(* Logix 5000 Rung export; software revision 20.03 *)

TYPE CONTROL_OUT_1 :
STRUCT
   TriggerEnable : BOOL;
   Trigger : BOOL;
   BufferResultsEnable : BOOL;
   InspectionResultsAck : BOOL;
   ExecuteCommand : BOOL;
   Reserved0_5 : BOOL;
   Reserved0_6 : BOOL;
   SetOffline : BOOL;
   Reserved_Byte1 : SINT;
   SetUserData : BOOL;
   Reserved2_1 : BOOL;
   ClearError : BOOL;
   ClearExposureComplete : BOOL;
   Reserved2_4 : BOOL;
   Reserved2_5 : BOOL;
   Reserved2_6 : BOOL;
   Reserved2_7 : BOOL;
   ExternalEvent0 : BOOL;
   ExternalEvent1 : BOOL;
   ExternalEvent2 : BOOL;
   ExternalEvent3 : BOOL;
   ExternalEvent4 : BOOL;
   ExternalEvent5 : BOOL;
   ExternalEvent6 : BOOL;
   ExternalEvent7 : BOOL;
   CommandID : INT;
   Reserved_Bytes6and7 : INT;
END_STRUCT
END_TYPE

TYPE INSIGHT_IN_1 :
STRUCT
   Status : STATUS_IN_1;
   InspectionResults : SINT[484];
END_STRUCT
END_TYPE

TYPE STATUS_IN_1 :
STRUCT
   TriggerReady : BOOL;
   TriggerAck : BOOL;
   Reserved0_2 : BOOL;
   AcqError : BOOL;
   OfflineReason0 : BOOL;
   OfflineReason1 : BOOL;
   OfflineReason2 : BOOL;
   Online : BOOL;
   Reserved1_0 : BOOL;
   InspectionCompleted : BOOL;
   ResultsBufferOverrun : BOOL;
   ResultsValid : BOOL;
   CommandExecuting : BOOL;
   CommandCompleted : BOOL;
   CommandFailed : BOOL;
   Error : BOOL;
   SetUserDataAck : BOOL;
   Reserved2_1 : BOOL;
   Reserved2_2 : BOOL;
   ExposureComplete : BOOL;
   JobPass : BOOL;
   TestRunReady : BOOL;
   Reserved2_6 : BOOL;
   Reserved2_7 : BOOL;
   ExternalEventAck0 : BOOL;
   ExternalEventAck1 : BOOL;
   ExternalEventAck2 : BOOL;
   ExternalEventAck3 : BOOL;
   ExternalEventAck4 : BOOL;
   ExternalEventAck5 : BOOL;
   ExternalEventAck6 : BOOL;
   ExternalEventAck7 : BOOL;
   ErrorID : INT;
   CommandResultCode : INT;
   CurrentJobID : INT;
   AcquisitionID : INT;
   InspectionID : INT;
   InspectionResultCode : INT;
END_STRUCT
END_TYPE

TYPE INSIGHT_OUT_1 :
STRUCT
   Control : CONTROL_OUT_1;
   UserData : SINT[488];
END_STRUCT
END_TYPE

VAR_GLOBAL   (* controller tags *)
   insight1_in : INSIGHT_IN_1;
   insight1_out : INSIGHT_OUT_1;
END_VAR

PROGRAM MainProgram

ROUTINE MainRoutine   (* ladder *)
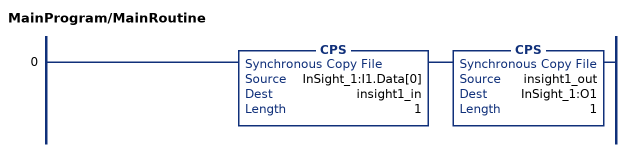
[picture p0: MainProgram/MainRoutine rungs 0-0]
   0: CPS(InSight_1:I1.Data[0],insight1_in,1)CPS(insight1_out,InSight_1:O1,1);
END_ROUTINE
END_PROGRAM
